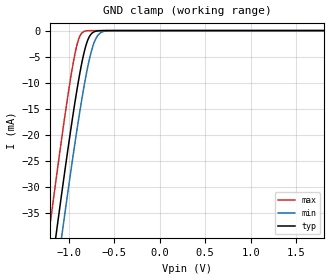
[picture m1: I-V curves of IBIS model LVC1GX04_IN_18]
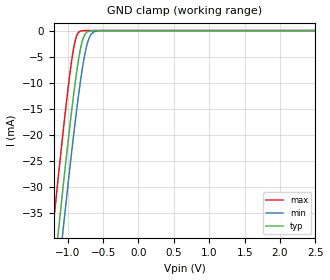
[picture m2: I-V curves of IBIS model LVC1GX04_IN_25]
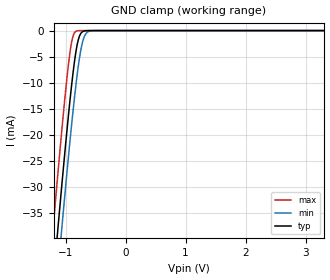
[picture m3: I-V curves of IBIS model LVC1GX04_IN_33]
| TEXAS INSTRUMENTS INCORPORATED
| Standard Linear and Logic Group
| IBIS Model of SN74LVC1GX04
| Crystal Oscillator Driver
| This file contains package information for the following:
|  SOT 6-pin (DBV) package as [Component] LVC1GX04_DBV
|  SOT 6-pin (DCK) package as [Component] LVC1GX04_DCK
| This device can be powered at the following Vccs:
|  1.8 volt Vcc
|  2.5 volt Vcc
|  3.3 volt Vcc
|  5 volt Vcc
| This file provides unique models under the [Model Selector] for each Vcc.
| For operation at a specific Vcc, select the appropriate model after each
| [Model Selector] keyword.
[IBIS Ver]   3.2
[Comment char]  |_char
[File Name]   sn74lvc1gx04.ibs
[File Rev]   1.1 | d_die
[Date]   May 04, 2004
[Source]   Data created from TI-SPICE simulations at TI-SLL.
[Notes]   The following is an IBIS list for the LVC1GX04.
   Please contact sllibis@ti.com with questions and
   comments concerning SLL IBIS models.
   - FILE REV HISTORY
   - 1.1 Release IBIS file on 05/04/04
   - Due to the fact that the Device is 5.5-V Input tolarent,
   the pulldown model has some Non-Monotonic Warnings.
   - Power clamp data deleted as there is no power-clamp diode.
[Disclaimer] Property of Texas Instruments Incorporated.  Unauthorized
   reproduction and/or distribution is strictly prohibited.
   This product is protected under copyright law.
   Created  2003, (C) Copyright  2003, Texas Instruments
   Incorporated, All Rights Reserved
   UNLESS THERE IS A SIGNED, WRITTEN AGREEMENT TO THE
   CONTRARY, TEXAS INSTRUMENTS (TI) IS PROVIDING THE IBIS
   MODELS  AND WITHOUT ANY WARRANTY, EXPRESSED OR
   IMPLIED.  TI assumes no liability for:
   1) the accuracy of the IBIS models provided to your
   company;
   2) the proper functioning of these IBIS Models in your
   design or for any resulting applications; or
   3) infringement of patents, copyrights or intellectual
   property rights resulting from your use of these IBIS
   models.
   TI provides IBIS Models as a service to our customers.
   You and your company shall not distribute, sell or give
   these models to anyone else without prior written
   permission from TI.
   TI reserves the right to make changes to our products or
   to discontinue any semiconductor product or service
   without notice, and advises our customers to obtain the
   latest version of relevant information to verify, before
   placing orders, that the information being relied on is
   current.
   Please be aware that your receipt and use of the IBIS
   information provided shall serve as acceptance of these
   terms and conditions.  If you do not accept these terms,
   you should return or destroy the IBIS models and any
   other accompanying information immediately.
| Component LVC1GX04_DBV 6-pin SOT
[Component]   LVC1GX04_DBV
[Manufacturer]   Texas Instruments, Inc.
[Package]
|   typ   min   max
R_pkg   2.500e-02   1.900e-02   3.700e-02
L_pkg   1.524e-09   1.260e-09   1.751e-09
C_pkg   2.450e-13   1.980e-13   2.640e-13
[Pin]   signal_name   model_name   R_pin   L_pin   C_pin
1   NC   NC   2.100e-02   1.405e-09   2.460e-13
2   GND   GND   3.700e-02   1.751e-09   2.630e-13
3   X1   LVC1GX04_IN   2.600e-02   1.493e-09   2.470e-13
4   X2   LVC1GX04_OUT   1.900e-02   1.620e-09   2.640e-13
5   VCC   POWER   2.400e-02   1.260e-09   1.980e-13
6   Y   LVC1GX04_OUT   2.100e-02   1.617e-09   2.500e-13
| Component LVC1GX04_DCK 6-pin SOT
[Component]   LVC1GX04_DCK
[Manufacturer]   Texas Instruments, Inc.
[Package]
|   typ   min   max
R_pkg   1.400e-02   1.100e-02   2.100e-02
L_pkg   9.480e-10   7.840e-10   1.103e-09
C_pkg   1.910e-13   1.670e-13   2.050e-13
[Pin]   signal_name   model_name   R_pin   L_pin   C_pin
1   NC   NC   1.300e-02   9.840e-10   1.960e-13
2   GND   GND   2.100e-02   1.103e-09   2.050e-13
3   X1   LVC1GX04_IN   1.100e-02   9.980e-10   1.970e-13
4   X2   LVC1GX04_OUT   1.300e-02   9.040e-10   1.900e-13
5   VCC   POWER   1.500e-02   7.840e-10   1.670e-13
6   Y   LVC1GX04_OUT   1.200e-02   9.160e-10   1.950e-13
| Model LVC1GX04_IN
[Model Selector]   LVC1GX04_IN
LVC1GX04_IN_18   1.8 volt Vcc
LVC1GX04_IN_25   2.5 volt Vcc
LVC1GX04_IN_33   3.3 volt Vcc
LVC1GX04_IN_50   5 volt Vcc
| Model LVC1GX04_OUT
[Model Selector]   LVC1GX04_OUT
LVC1GX04_OUT_18   1.8 volt Vcc
LVC1GX04_OUT_25   2.5 volt Vcc
LVC1GX04_OUT_33   3.3 volt Vcc
LVC1GX04_OUT_50   5 volt Vcc
| Models and submodels in the file (8): LVC1GX04_IN_18 (Input), LVC1GX04_IN_25 (Input), LVC1GX04_IN_33 (Input), LVC1GX04_IN_50 (Input), LVC1GX04_OUT_18 (Output), LVC1GX04_OUT_25 (Output), LVC1GX04_OUT_33 (Output), LVC1GX04_OUT_50 (Output)
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[Model]   LVC1GX04_IN_18
Model_type  Input
Vinl=0.5775
Vinh=1.2675
| variable   typ   min   max
C_comp   5.91pF   3.49pF   6.84pF
[Temperature Range]   40   100   -40
| Ambient temperature   25   85   -40
[Voltage range]   1.8   1.65   1.95
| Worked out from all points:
|   GND clamp passes 1 mA (typ) near -0.77 V on its own axis
[GND Clamp]
| LVC1GX04_IN_18
|   Voltage   I(typ)   I(min)   I(max)
-5.5V     -655.2mA   -662.2mA   -646.6mA
-1.215V   -49.6mA    -57.88mA   -38.96mA
-1.135V   -39.07mA   -47.36mA   -28.42mA
-1.075V   -31.35mA   -39.6mA    -20.75mA
-1.055V   -28.82mA   -37.05mA   -18.27mA
-955mV    -16.68mA   -24.66mA   -6.874mA
-885mV    -9.098mA   -16.55mA   -1.486mA
-825mV    -3.922mA   -10.26mA   -137.1uA
-780mV    -1.472mA   -6.227mA   -17.15uA
-715mV    -205.4uA   -2.128mA   -808.5nA
-650mV    -22.01uA   -443.9uA   -37.93nA
1.8V      3.326pA    6.142pA    3.026pA
[Model]   LVC1GX04_IN_25
Model_type  Input
Vinl=0.7
Vinh=1.7
| variable   typ   min   max
C_comp   6.22pF   4.01pF   7.75pF
[Temperature Range]   40   100   -40
| Ambient temperature   25   85   -40
[Voltage range]   2.5   2.3   2.7
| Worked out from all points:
|   GND clamp passes 1 mA (typ) near -0.77 V on its own axis
[GND Clamp]
| LVC1GX04_IN_25
|   Voltage   I(typ)   I(min)   I(max)
-5.5V     -655.2mA   -662.2mA   -646.6mA
-1.215V   -49.6mA    -57.88mA   -38.96mA
-1.14V    -39.72mA   -48.01mA   -29.07mA
-1.12V    -37.12mA   -45.41mA   -26.48mA
-1.08V    -31.98mA   -40.25mA   -21.38mA
-1.06V    -29.44mA   -37.69mA   -18.89mA
-960mV    -17.26mA   -25.26mA   -7.377mA
-890mV    -9.597mA   -17.1mA    -1.734mA
-785mV    -1.671mA   -6.635mA   -21.67uA
-720mV    -242.5uA   -2.354mA   -1.023uA
-650mV    -22.01uA   -443.9uA   -37.93nA
2.5V      4.713pA    7.577pA    4.389pA
[Model]   LVC1GX04_IN_33
Model_type  Input
Vinl=0.8
Vinh=2.0
| variable   typ   min   max
C_comp   6.34pF   4.26pF   7.86pF
[Temperature Range]   40   100   -40
| Ambient temperature   25   85   -40
[Voltage range]   3.3   3   3.6
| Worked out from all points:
|   GND clamp passes 1 mA (typ) near -0.77 V on its own axis
[GND Clamp]
| LVC1GX04_IN_33
|   Voltage   I(typ)   I(min)   I(max)
-5.5V     -655.2mA   -662.2mA   -646.6mA
-1.225V   -50.93mA   -59.21mA   -40.3mA
-1.145V   -40.37mA   -48.66mA   -29.72mA
-1.12V    -37.12mA   -45.41mA   -26.48mA
-1.08V    -31.98mA   -40.25mA   -21.38mA
-1.06V    -29.44mA   -37.69mA   -18.89mA
-965mV    -17.84mA   -25.87mA   -7.89mA
-885mV    -9.098mA   -16.55mA   -1.486mA
-780mV    -1.472mA   -6.227mA   -17.15uA
-715mV    -205.4uA   -2.128mA   -808.5nA
-640mV    -15.53uA   -338.1uA   -23.69nA
3.3V      6.304pA    9.258pA    5.93pA
